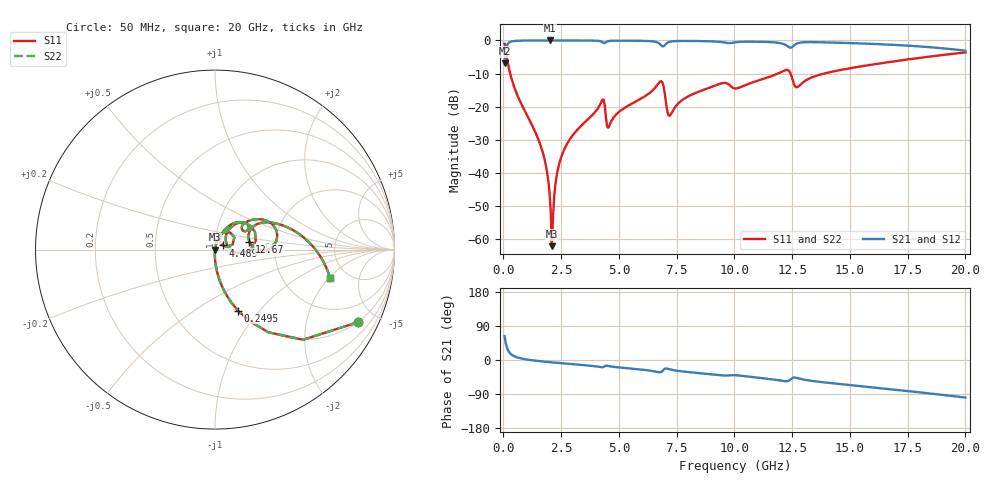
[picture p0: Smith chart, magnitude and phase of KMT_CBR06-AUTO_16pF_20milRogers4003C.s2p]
! Data measured by Modelithics Inc. support@modelithics.com 813-866-6335
! KEMET CBR06-AUTO 16pF, Pad Width= 0.851mm, Pad Length= 0.64mm, Pad Gap= 0.62mm, 20mil Rogers 4003C substrate Data, January 2022
# hz S ma R 50
! 2 Port Network Data from SP1.SP block
! freq  magS11  angS11  magS21  angS21  magS12  angS12  magS22  angS22
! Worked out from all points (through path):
!   401 points, 50 MHz to 20 GHz, reference 50 ohm
!   highest |S21| = -0.01 dB at 1.995 GHz (marker M1); lowest = -6.9 dB at 50 MHz (marker M2)
!   group delay of S21, straight-line fit = 14.1 ps
!   lowest |S11| = -62.1 dB at 2.095 GHz (marker M3), VSWR 1.00, Z = 50.1 - j0.0354 ohm
!   |S11| at or under -10 dB: 291.2 MHz to 11.89 GHz (11.59 GHz wide, 190 % of centre); 12.43 GHz to 13.88 GHz (1.456 GHz wide, 11.1 % of centre)
!   |S22| runs from -62.1 to -1.0 dB; largest |S21 - S12| = 0
!   S11 on the Smith chart (normalised r, x): 50 MHz: 0.99, -3.93; 249.5 MHz: 0.99, -0.78; 4.489 GHz: 1.09, +0.05; 12.67 GHz: 1.47, +0.13; 20 GHz: 3.68, -2.03
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5e7  0.892 -27.0  0.4517 63.0  0.4517 63.0  0.892 -27.0
2.495e8  0.3637 -69.4  0.9311 20.6  0.9311 20.6  0.3637 -69.4
6.98375e8  0.1252 -84.7  0.9917 5.1  0.9917 5.1  0.1252 -84.7
1.646e9  0.0236 -92.0  0.999 -3.5  0.999 -3.5  0.0236 -92.0
1.895375e9  0.009964 -91.1  0.9992 -5.1  0.9992 -5.1  0.009964 -91.1
1.995125e9  0.005046 -87.5  0.9992 -5.6  0.9992 -5.6  0.005046 -87.5
2.094875e9  0.0007818 -26.8  0.9992 -6.2  0.9992 -6.2  0.0007818 -26.8
2.34425e9  0.01079 78.2  0.9991 -7.6  0.9991 -7.6  0.01079 78.2
2.493875e9  0.01702 78.8  0.9989 -8.4  0.9989 -8.4  0.01702 78.8
3.391625e9  0.05258 75.5  0.9972 -13.1  0.9972 -13.1  0.05258 75.5
4.2395e9  0.1183 56.6  0.9641 -19.2  0.9641 -19.2  0.1183 56.6
4.488875e9  0.04992 27.6  0.9627 -15.3  0.9627 -15.3  0.04992 27.6
6.73325e9  0.2284 39.7  0.9058 -32.5  0.9058 -32.5  0.2284 39.7
6.882875e9  0.2325 12.1  0.8132 -29.2  0.8132 -29.2  0.2325 12.1
7.232e9  0.07501 34.7  0.9599 -25.1  0.9599 -25.1  0.07501 34.7
8.429e9  0.1668 53.1  0.9785 -34.5  0.9785 -34.5  0.1668 53.1
1.0025e10  0.188 35.1  0.9347 -40.0  0.9347 -40.0  0.188 35.1
1.22195e10  0.3562 20.1  0.8524 -56.1  0.8524 -56.1  0.3562 20.1
1.266838e10  0.1962 12.7  0.8856 -46.9  0.8856 -46.9  0.1962 12.7
1.336662e10  0.2778 31.1  0.9422 -55.2  0.9422 -55.2  0.2778 31.1
1.670825e10  0.4719 11.1  0.8636 -76.8  0.8636 -76.8  0.4719 11.1
2e10  0.6592 -13.7  0.6992 -99.0  0.6992 -99.0  0.6592 -13.7
